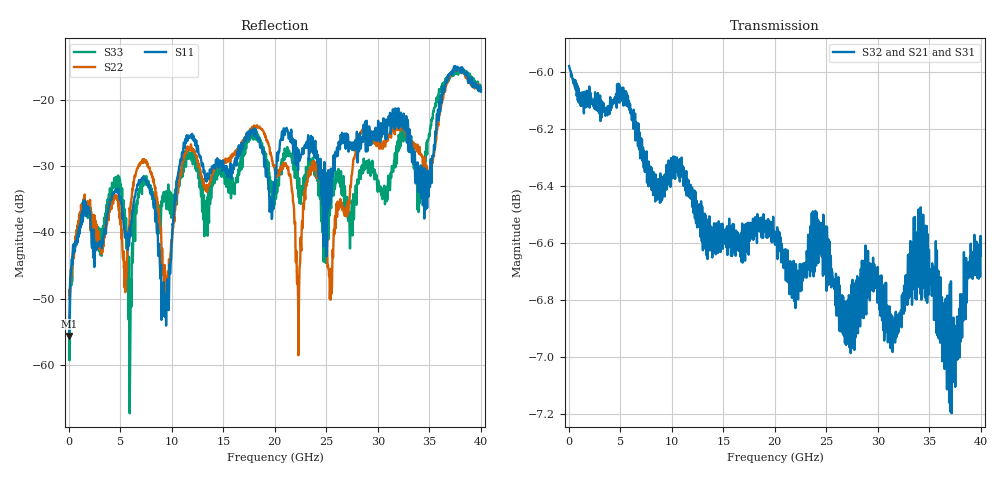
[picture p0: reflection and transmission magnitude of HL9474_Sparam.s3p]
! 1/15/2020 10:17:33 AM
! H:\PRODUCTION_DATA\9474\9474-PROTO1-01-15-2020.S3P
! CHANNEL.1
! TR.MEASUREMENT
! CORRECTED.DATA
# GHZ S RI R 50.0
! FREQ.GHZ  S11RE  S11IM  S12RE  S12IM  S13RE  S13IM
!  S21RE  S21IM  S22RE  S22IM  S23RE  S23IM
!  S31RE  S31IM  S32RE  S32IM  S33RE  S33IM
!; PortSelection: Port_123
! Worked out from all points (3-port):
!   1143 points, 35 MHz to 40.01 GHz, reference 50 ohm
!   strongest paths, dB at 35 MHz, 10.01 GHz, 20.02 GHz, 30.03 GHz, 40.01 GHz:
!     S32: -6.0, -6.3, -6.6, -6.8, -6.6
!     S21: -6.0, -6.3, -6.5, -6.8, -6.5
!     S31: -6.1, -6.5, -6.5, -6.8, -6.8
!   lowest |S11| = -55.6 dB at 35 MHz (marker M1), VSWR 1.00, Z = 50.1 + j0.0964 ohm
!   |S11| at or under -10 dB: start of sweep to end of sweep
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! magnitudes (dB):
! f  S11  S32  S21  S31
! 35 MHz  -55.6  -6.0  -6.0  -6.1
! 4.62 GHz  -33.8  -6.1  -6.2  -6.2
! 5.915 GHz  -39.3  -6.1  -6.2  -6.2
! 7.315 GHz  -31.8  -6.3  -6.4  -6.4
! 9.275 GHz  -51.9  -6.4  -6.3  -6.4
! 11.48 GHz  -25.6  -6.4  -6.4  -6.6
! 20.02 GHz  -34.1  -6.6  -6.5  -6.5
! 25.38 GHz  -35.7  -6.7  -6.7  -6.7
! 28.35 GHz  -27.4  -6.7  -6.9  -7.1
! 40.01 GHz  -18.8  -6.6  -6.5  -6.8
